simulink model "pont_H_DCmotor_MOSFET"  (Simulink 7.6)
settings: Solver=ode23tb  StartTime=0.0  StopTime=4.5  MaxStep=0.02  RelTol=1e-4
InitFcn:
  | clc
  | clear all
  | close all
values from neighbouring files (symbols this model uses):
  A = [1+j -(1-j);1 -2/(1-j)]    [systeme_AX_B_phaseurs.m]
  N = 50;')    [Prog_callbacks.m]    (also in _startup.m = 0.001'))
undefined symbols (not defined in the file or in its folder): constant, Torque
libraries: powerlib x12

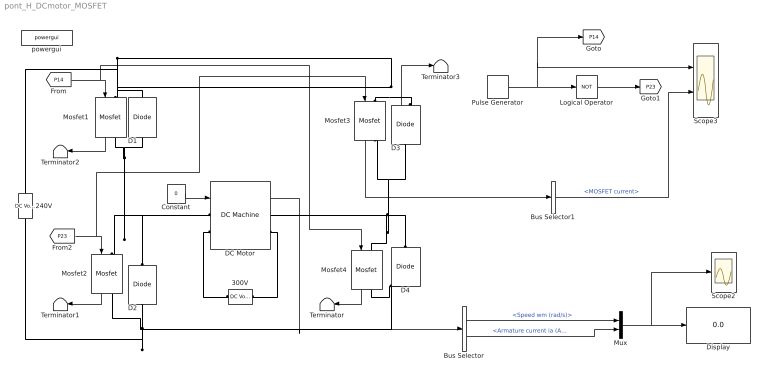
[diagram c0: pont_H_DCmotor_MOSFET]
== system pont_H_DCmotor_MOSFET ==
  240V : powerlib/Electrical Sources/DC Voltage Source  DialogController=POWERSYS.PowerSysDialog  SystemSampleTime=-1  Amplitude=240  Measurements=None
  300V : powerlib/Electrical Sources/DC Voltage Source  DialogController=POWERSYS.PowerSysDialog  SystemSampleTime=-1  Amplitude=300  Measurements=None
  Bus Selector : BusSelector  OutputSignals=Speed wm (rad/s),Armature current ia (A)
  Bus Selector1 : BusSelector  OutputSignals=MOSFET current
  Constant : Constant  Value=0
  D1 : powerlib/Power Electronics/Diode  DialogController=POWERSYS.PowerSysDialog  SystemSampleTime=-1  Ron=0.001  Lon=0  Vf=0.8  IC=0  UseSnubber=off  Rs=inf  Cs=0  Measurements=off
  D2 : powerlib/Power Electronics/Diode  DialogController=POWERSYS.PowerSysDialog  SystemSampleTime=-1  Ron=0.001  Lon=0  Vf=0.8  IC=0  UseSnubber=off  Rs=inf  Cs=0  Measurements=off
  D3 : powerlib/Power Electronics/Diode  DialogController=POWERSYS.PowerSysDialog  SystemSampleTime=-1  Ron=0.001  Lon=0  Vf=0.8  IC=0  UseSnubber=off  Rs=inf  Cs=0  Measurements=on
  D4 : powerlib/Power Electronics/Diode  DialogController=POWERSYS.PowerSysDialog  SystemSampleTime=-1  Ron=0.001  Lon=0  Vf=0.8  IC=0  UseSnubber=off  Rs=inf  Cs=0  Measurements=off
  DC Motor : powerlib/Machines/DC Machine  DialogController=POWERSYS.PowerSysDialog  SystemSampleTime=-1  PresetModel=01: 5HP 240V 1750RPM Field:300V  MechanicalLoad=Torque TL  FieldType=Wound  ShowDetailedParameters=on  RLa=[2.581 0.028]  RLf=[281.3 156]  Laf=0.9483  MachineConstant=Torque constant (N.m/A)  Ke=1.8  Kt=1.8  J=0.02215  Bm=0.002953  Tf=0.5161  w0=0.001  Ifinit=1.06647707074298  TsPowergui=0  TsBlock=-1
  Display : Display
  Logical Operator : Logic  Operator=NOT  AllPortsSameDT=off  OutDataTypeStr=boolean
  "Mosfet1 " : powerlib/Power Electronics/Mosfet  DialogController=POWERSYS.PowerSysDialog  SystemSampleTime=-1  Ron=0.1  Lon=0  Rd=0.01  Vfd=0  IC=0  Rs=1e5  Cs=inf  Measurements=on
  Mosfet2 : powerlib/Power Electronics/Mosfet  DialogController=POWERSYS.PowerSysDialog  SystemSampleTime=-1  Ron=0.1  Lon=0  Rd=0.01  Vfd=0  IC=0  Rs=1e5  Cs=inf  Measurements=on
  Mosfet3 : powerlib/Power Electronics/Mosfet  DialogController=POWERSYS.PowerSysDialog  SystemSampleTime=-1  Ron=0.1  Lon=0  Rd=0.01  Vfd=0  IC=0  Rs=1e5  Cs=inf  Measurements=on
  Mosfet4 : powerlib/Power Electronics/Mosfet  DialogController=POWERSYS.PowerSysDialog  SystemSampleTime=-1  Ron=0.1  Lon=0  Rd=0.01  Vfd=0  IC=0  Rs=1e5  Cs=inf  Measurements=on
  Mux : Mux  Inputs=2
  Pulse Generator : DiscretePulseGenerator  PulseType=Time based  Period=1  PulseWidth=80
  Scope2 : Scope
  Scope3 : Scope  NumInputPorts=2
  Terminator{,1..3} (4 alike) : Terminator
  powergui : powerlib/powergui  SystemSampleTime=-1  SimulationMode=Continuous  SampleTime=20e-6  frequency=60  SPID=off  DisableSnubberDevices=off  DisableRonSwitches=off  DisableVfSwitches=off  SwTol=0  Interpol=off  frequencyindice=0  echomessages=off  HookPort=off  DisplayEquations=off  FunctionMessages=off  EnableUseOfTLC=off  x0status=blocks  RestoreLinks=warning  ResistiveCurrentMeasurement=off  Frange=[0:2:500]  Ylog=off  Xlog=on  ShowGrid=off  save=off  variable=ZData  ZoomFFT=on  StartTime=0.0  cycles=1  DisplayStyle=1  fundamental=60  FreqAxis=off  MaxFrequency=1000  frequencyindicesteady=1  RmsSteady=1  display=off  Ts=0  methode=off
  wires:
  [P14] -> "Mosfet1 "/1, Mosfet4/1
  Pulse Generator/1 -> Logical Operator/1, [P14], Scope3/1
  Logical Operator/1 -> [P23]
  [P23] -> Mosfet2/1, Mosfet3/1
  Mosfet3/1 -> Bus Selector1/1
  Bus Selector/1 -> Mux/1  "<Speed wm (rad/s)>"
  Bus Selector/2 -> Mux/2  "<Armature current ia (A)>"
  Mux/1 -> Display/1, Scope2/1
  Bus Selector1/1 -> Scope3/2  "<MOSFET current>"
  Constant/1 -> DC Motor/1
  DC Motor/1 -> Bus Selector/1
  Mosfet4/1 -> Terminator/1
  Mosfet2/1 -> Terminator1/1
  "Mosfet1 "/1 -> Terminator2/1
  D3/1 -> Terminator3/1
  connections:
  Mosfet2/LConn1 -- D2/RConn1 -- D1/LConn1 -- "Mosfet1 "/RConn1 -- DC Motor/LConn1
  D4/RConn1 -- Mosfet4/LConn1 -- Mosfet3/RConn1 -- D3/LConn1 -- DC Motor/RConn1
  Mosfet3/LConn1 -- D1/RConn1 -- "Mosfet1 "/LConn1 -- 240V/RConn1 -- D3/RConn1
  240V/LConn1 -- D4/LConn1 -- Mosfet4/RConn1 -- D2/LConn1 -- Mosfet2/RConn1
  300V/RConn1 -- DC Motor/LConn2
  DC Motor/RConn2 -- 300V/LConn1
